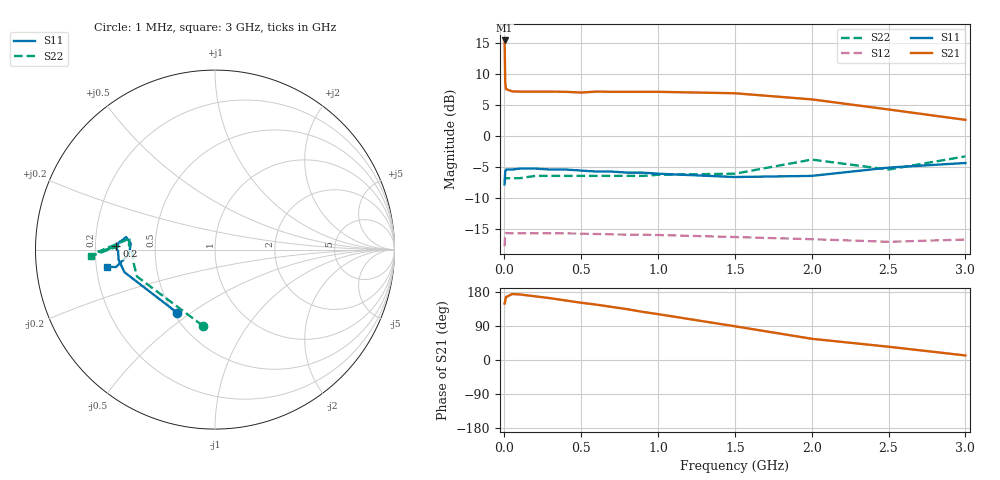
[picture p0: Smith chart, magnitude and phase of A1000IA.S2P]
!  MSA1000 S PARAMETERS
!  Id=325 mA  LAST UPDATED 07-27-92
# ghz s ma r 50
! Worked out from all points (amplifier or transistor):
!   18 points, 1 MHz to 3 GHz, reference 50 ohm
!   highest |S21| = 15.5 dB at 1 MHz (marker M1)
!   |S21| within 3 dB of that: start of sweep to 2.773 MHz
!   unconditionally stable (mu >= 1): 4.744 MHz to 1.572 GHz
!   at 50 MHz: K = 1.17, MAG = 9.0 dB, |S12| = -15.7 dB
!   at 600 MHz: K = 1.16, MAG = 9.1 dB, |S12| = -15.8 dB
!   at 3 GHz: K = 0.50, MSG = 9.7 dB, |S12| = -16.7 dB
!   S11 on the Smith chart (normalised r, x): 1 MHz: 0.52, -0.44; 200 MHz: 0.29, +0.02; 3 GHz: 0.24, -0.07
0.001  0.41 -121.0  5.95 149.0  0.13 22.0  0.43 -99.0
0.005  0.52 -166.0  2.73 156.0  0.164 6.0  0.46 -161.0
0.01  0.54 -174.0  2.41 166.0  0.166 3.0  0.46 -171.0
0.05  0.54 -179.0  2.31 174.0  0.165 0.0  0.46 -178.0
0.1  0.55 179.0  2.3 173.0  0.165 -1.0  0.46 -179.0
0.2  0.55 178.0  2.3 168.0  0.165 -1.0  0.48 177.0
0.3  0.54 177.0  2.3 163.0  0.165 -2.0  0.48 176.0
0.4  0.54 176.0  2.29 157.0  0.165 -3.0  0.48 176.0
0.5  0.53 175.0  2.26 151.0  0.164 -3.0  0.48 176.0
0.6  0.52 175.0  2.3 146.0  0.163 -4.0  0.48 174.0
0.7  0.52 174.0  2.29 140.0  0.162 -4.0  0.48 174.0
0.8  0.51 174.0  2.29 134.0  0.161 -5.0  0.48 173.0
0.9  0.51 173.0  2.29 127.0  0.161 -5.0  0.48 173.0
1  0.5 172.0  2.29 121.0  0.16 -5.0  0.49 172.0
1.5  0.47 176.0  2.23 89.0  0.154 -7.0  0.5 174.0
2  0.48 -177.0  1.99 56.0  0.148 -10.0  0.65 -179.0
2.5  0.56 -170.0  1.65 35.0  0.141 -1.0  0.54 178.0
3  0.61 -171.0  1.36 12.0  0.147 1.0  0.69 -177.0
